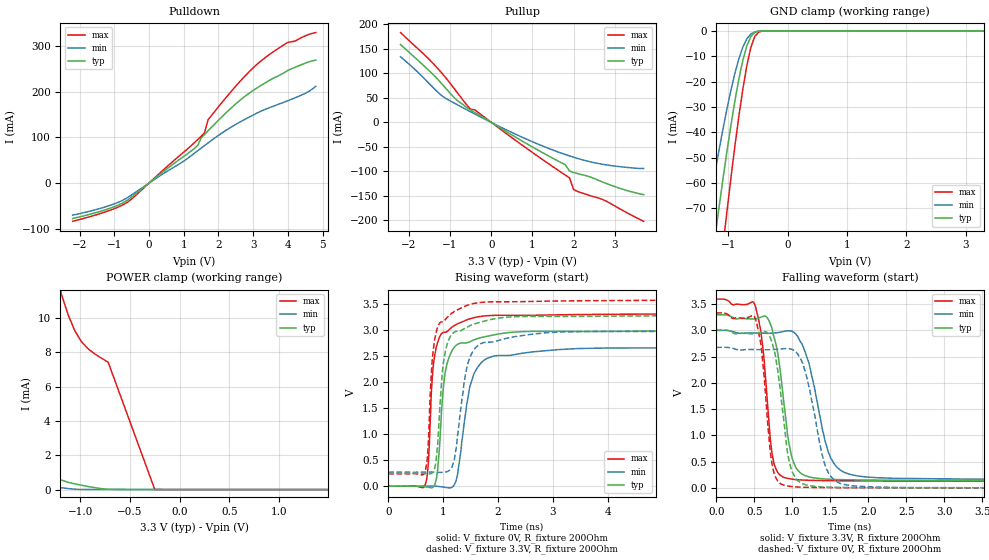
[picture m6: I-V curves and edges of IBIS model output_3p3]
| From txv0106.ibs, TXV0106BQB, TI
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|   io_3p3 Model
[Model]   output_3p3
Model_type   I/O
Polarity   Non-Inverting
Enable   Active-High
Vinl = 0.99
Vinh = 2.310
Vmeas = 1.65
Vref = 0
Cref = 0.2pF
Rref = 100000
|   typ   min   max
C_comp   1.540pF   1.379pF   1.785pF
| Where Nom  PVT is Nominal Process, 3.3V, 27C
|   Fast PVT is Strong Process,  3.6V, -40C
|   Slow PVT is Weak Process,   3.0V, 130C
[Voltage Range]   3.3   3   3.6
|Junction Temperature
[Temperature Range]   27   130   -40
[Pullup Reference]   3.3   3   3.6
[Pulldown Reference]   -0   0   0
[Power Clamp Reference]   3.3   3   3.6
[GND Clamp Reference]   0   0   0
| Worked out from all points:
|   slope of the pulldown table from 0 to 0.495 V, typ, clamps not added: 16.6 ohm
|   slope of the pullup table from 0 to 0.495 V, typ, clamps not added: 19.5 ohm
|   GND clamp passes 1 mA (typ) near -0.57 V on its own axis
|   POWER clamp passes 1 mA (typ) near -1.28 V on its own axis
|   falling waveform, V_fixture 3.3V, R_fixture 200Ohm: 20-80 % time 172ps typ, 259ps min, 126ps max; typ from 3.3 V to 0.136 V
|   rising waveform, V_fixture 0V, R_fixture 200Ohm: 20-80 % time 164ps typ, 251ps min, 133ps max; typ from 0 V to 3.01 V
|   rising waveform, V_fixture 3.3V, R_fixture 200Ohm: 20-80 % time 159ps typ, 234ps min, 133ps max; typ from 0.249 V to 3.3 V
|   falling waveform, V_fixture 0V, R_fixture 200Ohm: 20-80 % time 156ps typ, 226ps min, 119ps max; typ from 3.01 V to 0 V
[Pulldown]
|Voltage  I(typ)   I(min)   I(max)
-2.2V     -77.49mA   -70.09mA   -83.57mA
-1.2V     -57.03mA   -50.71mA   -61.53mA
-600mV    -36.29mA   -30.81mA   -40.77mA
1.3V      75.29mA    64.79mA    87.89mA
1.4V      82.22mA    70.58mA    95.02mA
1.5V      98.47mA    76.38mA    102.1mA
1.6V      106.4mA    82.14mA    110.4mA
1.7V      114.3mA    87.83mA    138.3mA
2.5V      173.3mA    128.4mA    212.1mA
3.1V      207.5mA    152.7mA    259mA
4V        246.5mA    180.1mA    307.7mA
4.8V      268.7mA    211.5mA    329mA
[GND Clamp]
|Voltage   I(typ)   I(min)   I(max)
-2.161V   -262.3mA   -202.7mA   -322.1mA
-1.357V   -106mA     -74.89mA   -142.8mA
-1.223V   -81.71mA   -56.2mA    -113.7mA
-1.156V   -69.99mA   -47.35mA   -99.38mA
-1.089V   -58.65mA   -38.91mA   -85.32mA
-1.022V   -47.76mA   -30.95mA   -71.6mA
-821mV    -19.13mA   -11.09mA   -33.81mA
-687mV    -5.965mA   -3.194mA   -13.85mA
-620mV    -2.337mA   -1.299mA   -6.642mA
-553mV    -661uA     -428.6uA   -2.22mA
-419mV    -23.68uA   -26.36uA   -69.53uA
3.3V      0A         0A         0A
[Pullup]
|Voltage   I(typ)   I(min)   I(max)
-2.2V     159mA      134mA      183.4mA
-1.5V     105.1mA    78.83mA    128.2mA
-1.1V     69.31mA    48.96mA    90.97mA
-800mV    43.18mA    35.13mA    58.25mA
-500mV    25.41mA    21.69mA    26.71mA
-400mV    20.12mA    17.28mA    25.86mA
600mV     -30.55mA   -24.35mA   -37.14mA
1.8V      -86.47mA   -65.6mA    -107.6mA
1.9V      -99.06mA   -68.4mA    -113.2mA
2V        -102.3mA   -71.08mA   -137mA
2.7V      -121.5mA   -85.41mA   -157.2mA
3.7V      -147.4mA   -94mA      -201.8mA
[POWER Clamp]
|Voltage  I(typ)   I(min)   I(max)
-2.328V   27.64mA    12.6mA     51.4mA
-2.261V   25.56mA    11.06mA    48.8mA
-1.993V   17.32mA    5.339mA    38.32mA
-1.792V   11.37mA    2.197mA    30.33mA
-1.524V   4.83mA     543.7uA    20.24mA
-1.39V    2.184mA    317.3uA    16.22mA
-1.256V   789.2uA    171.5uA    12.8mA
-1.189V   553.3uA    110.7uA    11.37mA
-988mV    253.5uA    9.565uA    8.617mA
-720mV    16.78uA    5.46uA     7.424mA
-251mV    1.565uA    3.275uA    7.297uA
1.491V    479.2nA    431.8nA    2.452uA
[Ramp]
R_load = 200
|   typ   min   max
dV/dt_r   1.805/0.164n   1.606/0.252n   1.999/0.133n
dV/dt_f   1.897/0.170n   1.708/0.258n   2.081/0.127n
[Falling Waveform]
V_fixture = 3.3V
V_fixture_min = 3V
V_fixture_max = 3.6V
R_fixture = 200Ohm
C_fixture = 0F
|   Time   V(typ)   V(min)   V(max)
0s        3.298V     2.999V     3.596V
500ps     3.219V     2.951V     3.516V
610ps     3.264V     2.947V     2.709V
690ps     3.197V     2.945V     1.32V
790ps     2.709V     2.954V     344.2mV
1.05ns    383mV      2.924V     156.8mV
1.45ns    166.6mV    812.7mV    137.8mV
1.86ns    151.5mV    226.6mV    133mV
4.99ns    137.9mV    159.9mV    127.1mV
200ns     135.8mV    152.5mV    126.5mV
[Rising Waveform]
V_fixture = 0V
V_fixture_min = 0V
V_fixture_max = 0V
R_fixture = 200Ohm
C_fixture = 0F
|   Time   V(typ)   V(min)   V(max)
0s        16.25uV    12.31uV    18.01uV
670ps     -8.901mV   -232.3uV   20.07mV
730ps     -19.66mV   576.7uV    460.3mV
840ps     17.85mV    2.495mV    2.474V
900ps     327.5mV    -3.165mV   2.766V
1.03ns    2.143V     -21.14mV   2.959V
1.19ns    2.653V     6.353mV    3.078V
1.55ns    2.808V     2.127V     3.235V
2.01ns    2.926V     2.512V     3.285V
200ns     3.008V     2.676V     3.332V
[Rising Waveform]
V_fixture = 3.3V
V_fixture_min = 3V
V_fixture_max = 3.6V
R_fixture = 200Ohm
C_fixture = 0F
|   Time   V(typ)   V(min)   V(max)
0s        248.9mV    268.8mV    238.6mV
670ps     241.8mV    270.1mV    283.7mV
720ps     237.6mV    270.8mV    668mV
830ps     302.4mV    272.2mV    2.701V
890ps     694.3mV    267.4mV    3.026V
1ns       2.343V     266.5mV    3.165V
1.12ns    2.855V     307mV      3.291V
1.47ns    3.076V     2.424V     3.487V
1.91ns    3.214V     2.774V     3.544V
200ns     3.298V     2.999V     3.596V
[Falling Waveform]
|Gnd
V_fixture = 0V
V_fixture_min = 0V
V_fixture_max = 0V
R_fixture = 200Ohm
C_fixture = 0F
| Time   V(typ)   V(min)   V(max)
0s        3.008V     2.676V     3.332V
510ps     2.94V      2.635V     3.24V
590ps     2.965V     2.633V     2.711V
680ps     2.945V     2.631V     1.17V
760ps     2.631V     2.636V     279mV
980ps     387.2mV    2.645V     27.88mV
1.31ns    25.83mV    1.28V      6.819mV
1.58ns    8.947mV    122.2mV    3.813mV
2.54ns    1.806mV    5.723mV    1.093mV
200ns     -223.9nV   -4.251nV   -23.11nV
